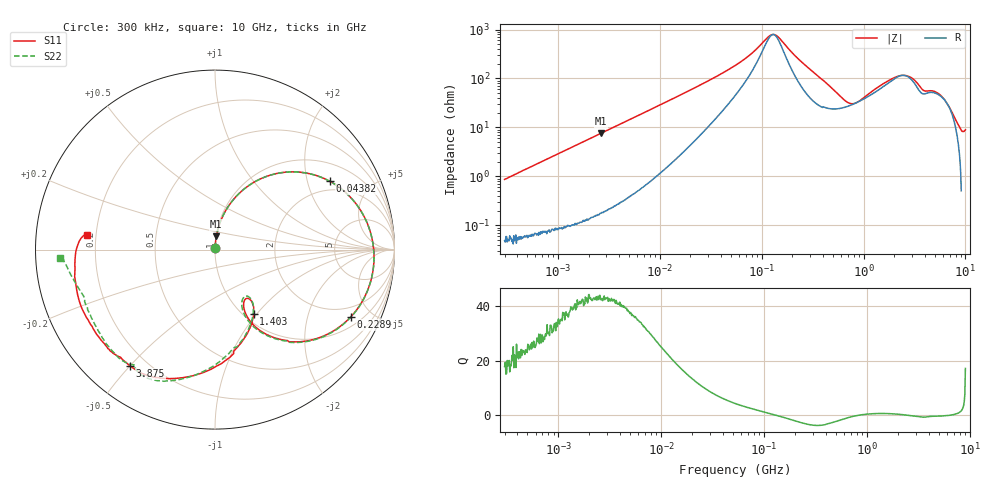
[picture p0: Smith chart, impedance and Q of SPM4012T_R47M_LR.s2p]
! S-Parameter Data Generated by TDK Corporation
! Copyright(C) 2019 TDK Corporation.
! All Rights Reserved.
! TDK P/N: SPM4012T-R47M-LR (Inductor)
! Property: L=470nH at 100kHz
! Size(LxWxT): 4.4x4.1x1.2mm
! Model Type: s2p (Touchstone File Format Version 1.0)
! Frequency: DC=Yes Start=0.3MHz Stop=10000MHz 802points Log-sweep
! Model Generated on Sep. 23, 2019
! Port Assignments:
!  1 ---@@@--- 2
! Applicable Conditions:
!  Temperature = 25 degC
!  DC Bias Current = 0 A
!  Small Signal Operation
! Terms and conditions regarding TDK Simulation Models
! (1)This simulation model is being provided solely for informational purposes. Please refer to the specifications of the products in terms of detailed characteristics of such products.
! (2)In no event shall TDK Corporation of any of its subsidiaries be liable for any loss or damage arising, directly or indirectly,
!  From any information contained in this simulation model, including, but not limited to loss or damages arising from any inaccuracies, omissions or errors in connection with such information.
! (3)Any and all copyrights on this simulation model are owned by TDK Corporation.
!  Duplication or redistribution of this simulation model without prior written permission from TDK Corporation is prohibited.
! (4)This simulation model is subject to any modification or change without any prior notice.
! (5)Neither TDK Corporation nor any of its subsidiaries shall make any warranty, express or implied,
!  Including but not limited to the correctness, implied warranties of merchantability and fitness for a particular purpose with respect to this simulation models.
! (6)The use of this simulation model shall be deemed to have consented to the terms and conditions hereof.
# Hz S MA R 50
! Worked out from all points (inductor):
!   801 points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, 300 kHz to 10 GHz, reference 50 ohm
!   read as one part in series: L = 460 nH near 318.3 kHz
!   highest Q = 43 at 2.631 MHz (marker M1), where L = 455 nH
!   self-resonance near 129.7 MHz
!   S11 on the Smith chart (normalised r, x): 300 kHz: 1.00, +0.02; 43.82 MHz: 1.63, +2.78; 228.9 MHz: 1.44, -3.75; 1.403 GHz: 1.11, -0.96; 3.875 GHz: 0.14, -0.50; 10 GHz: 0.16, +0.05
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300000  0.008494 85.9  0.9995 -0.5  0.9994 -0.5  0.008307 86.5
1713600  0.04853 85.8  0.9977 -2.8  0.9977 -2.8  0.04847 85.8
2631200  0.07408 84.3  0.9955 -4.3  0.9955 -4.3  0.07415 84.3
9671944  0.2612 72.3  0.955 -15.5  0.9551 -15.5  0.2612 72.2
2.441527e7  0.555 50.2  0.7817 -34.5  0.7817 -34.5  0.555 50.2
4.38171e7  0.7449 30.7  0.5443 -48.8  0.5443 -48.8  0.745 30.7
5.477226e7  0.7972 23.2  0.4395 -52.7  0.4395 -52.7  0.7973 23.1
1.291483e8  0.8881 -4.7  0.1119 -5.7  0.1119 -5.7  0.8881 -4.9
1.437797e8  0.8878 -8.4  0.1229 17.2  0.123 17.2  0.8877 -8.6
2.289088e8  0.8442 -26.4  0.3249 44.1  0.3249 44.1  0.8439 -26.8
3.126428e8  0.759 -40.4  0.4941 35.5  0.4942 35.5  0.7583 -40.9
4.448526e8  0.599 -55.5  0.6506 18.5  0.6507 18.4  0.5968 -56.1
6.656121e8  0.3989 -64.4  0.734 -5.1  0.7341 -5.1  0.3917 -65.7
9.560117e8  0.3236 -57.2  0.699 -27.3  0.699 -27.3  0.3099 -57.5
1.403063e9  0.4164 -58.9  0.5605 -51.0  0.5606 -51.0  0.3942 -57.2
1.767019e9  0.5162 -71.1  0.4365 -62.9  0.4366 -62.9  0.4927 -68.7
2.756092e9  0.7311 -103.2  0.2624 -62.9  0.2624 -62.9  0.7287 -102.1
3.874538e9  0.8013 -126.1  0.2861 -65.0  0.2861 -65.0  0.7972 -123.5
5.099159e9  0.8088 -134.0  0.2484 -79.2  0.2485 -79.2  0.8074 -130.7
6.333834e9  0.8101 -143.3  0.2353 -91.9  0.2354 -92.0  0.7921 -145.4
8.09931e9  0.7961 -169.1  0.2025 -114.7  0.2026 -114.8  0.8046 -167.7
1e10  0.7189 173.5  0.1522 -128.6  0.1523 -128.8  0.8637 -176.9
